(*
xml 存n行，每行4个参数，bool-可用位vaild、bool-输出位状态、bool-正反向输出标记位、lreal-节点坐标
使用METH进行调用，以实现区分功能， 以及少点高速性能。运行一次最多8个点。
.RUN() 一次加载全部数据，不支持中途改值
*)

FUNCTION_BLOCK FB_EL5131_SingleCycle
VAR CONSTANT
	{attribute 'displaymode':='hex'}
	cMaxCounterValue										: 	UDINT := 4294967295;
END_VAR
VAR_INPUT
	{attribute 'hide'} // 尝试隐藏该变量
	nDistWindow												:	UINT := 5;
	stEl5131												:	REFERENCE TO ST_EL5131;
	rScaleFactor      										: 	LREAL := 1; // 分子/分母
	{attribute 'displaymode':='bin'}
	OutputOption											:	USINT := 2#0000_0001; // chn 1 output
	InputOption												:	REFERENCE TO ST_EL5131_Setting;
END_VAR
VAR_OUTPUT
	bBusy													:	BOOL;
	bDone													:	BOOL;
	bError													:	BOOL;
	nErrId													:	UDINT;
	sErr													:	STRING;
	bInited													:	BOOL;
END_VAR
VAR
	{attribute 'hide'}
	_nMem													:	WORD;// bit 0 / 1 /2
	{attribute 'hide'}
	_pControOutput											:	POINTER TO ST_ENC_Control_Output_Channel;
	{attribute 'hide'}
	i														:	INT;
	{attribute 'hide'}
	_CamData												:	FB_MEM_TO_DATA_ST_EL5131_CamData;	
	{attribute 'hide'}
	_nNum													:	USINT;
	{attribute 'hide'}
	_tLastDurationDelay										:	TON :=(PT:= T#0S);
	{attribute 'hide'}
	nLastCounterValue										:	UDINT;
	{attribute 'hide'}
	_nTempLint												:	LINT;
	{attribute 'hide'}
	bForward												:	BOOL;
	{attribute 'hide'}
	bBackward												:	BOOL;
END_VAR

METHOD Cyclic : BOOL
VAR_INPUT
END_VAR
IF NOT __ISVALIDREF(stEl5131)
THEN
	RETURN;
END_IF
IF NOT _nMem.2
THEN 
	_nMem.2											:= TRUE;
	nLastCounterValue								:= stEl5131.PdoToPlc.Counter_value;
END_IF
bForward											:= FALSE;
bBackward											:= FALSE;
IF nLastCounterValue <> stEl5131.PdoToPlc.Counter_value
THEN 
	IF stEl5131.PdoToPlc.Counter_value > nLastCounterValue
	THEN 
		bForward									:= TRUE;
		bBackward									:= FALSE;
	END_IF
	IF stEl5131.PdoToPlc.Counter_value < nLastCounterValue
	THEN 
		bForward									:= FALSE;
		bBackward									:= TRUE;
	END_IF
	
	nLastCounterValue								:= stEl5131.PdoToPlc.Counter_value;
END_IF
END_METHOD

METHOD Init : BOOL
VAR_INPUT
	bExecute		:	BOOL;
END_VAR
Init														:= TRUE;
bInited														:= FALSE;
IF bExecute 
THEN
	IF NOT __ISVALIDREF(stEl5131)
	OR NOT (OutputOption.0 OR OutputOption.1)
	OR NOT __ISVALIDREF(InputOption)
	THEN 
		bBusy 												:= FALSE;
		bDone												:= FALSE;
		bError												:= TRUE;
		nErrId.0											:= TRUE;
		sErr												:= 'FB_EL5131_SingleCycle | FB_INPUT is not valid';
		RETURN;
	END_IF

	bBusy 													:= FALSE;
	bDone													:= FALSE;
	bError													:= FALSE;
	nErrId													:= 0;
	sErr													:= '';
	_nMem													:= 0;
	IF OutputOption.0 
	THEN 
		_pControOutput 										:= ADR(stEl5131.PlcToPdo.Contro_OutputChn1);
	END_IF							
	IF NOT OutputOption.0 
	AND OutputOption.1
	THEN 
		_pControOutput 										:= ADR(stEl5131.PlcToPdo.Contro_OutputChn2);
	END_IF
	_pControOutput^.Control.Enable_thresholds_output		:= TRUE;
	_pControOutput^.Control.Disalbe_thresholds_ccw			:= TRUE; // 在RUN 中根据情况再给false
	_pControOutput^.Control.Disalbe_thresholds_cw			:= TRUE; // 在RUN 中根据情况再给false
	_pControOutput^.Control.Set_tristate					:= InputOption.SetTristate;
	bInited													:= TRUE;
	Init													:= FALSE;
	
END_IF
END_METHOD

// 禁止模块输出
METHOD Reset : BOOL
VAR_INPUT
	bExecute		:	BOOL;
END_VAR
Reset														:= TRUE;
IF bExecute 
THEN 
	IF NOT __ISVALIDREF(stEl5131)
	OR NOT (OutputOption.0 OR OutputOption.1)
	OR NOT __ISVALIDREF(InputOption)
	THEN 
		bBusy 												:= FALSE;
		bDone												:= FALSE;
		bError												:= TRUE;
		nErrId.0											:= TRUE;
		sErr												:= 'FB_EL5131_SingleCycle | FB_INPUT is not valid';
		RETURN;
	END_IF
	// reset
	bBusy 													:= FALSE;
	bDone													:= FALSE;
	bError													:= FALSE;
	nErrId													:= 0;
	sErr													:= '';
	_nMem													:= 0;
	IF OutputOption.0 
	THEN 
		_pControOutput 										:= ADR(stEl5131.PlcToPdo.Contro_OutputChn1);
	END_IF
	IF NOT OutputOption.0 
	AND OutputOption.1
	THEN 
		_pControOutput 										:= ADR(stEl5131.PlcToPdo.Contro_OutputChn2);
	END_IF
	_pControOutput^.Control.Enable_thresholds_output		:= FALSE;
	_pControOutput^.Control.Disalbe_thresholds_ccw			:= TRUE;
	_pControOutput^.Control.Disalbe_thresholds_cw			:= TRUE;
	_pControOutput^.Control.Set_tristate					:= InputOption.SetTristate;
	bInited													:= FALSE;
	Reset													:= FALSE;
END_IF
END_METHOD

METHOD Run : BOOL
VAR_INPUT
	bExecute												:	BOOL;
	pstEL5131_CamData										:	POINTER TO ST_EL5131_CamData;
	nSize													:	ULINT;
END_VAR
Run															:= TRUE;
IF bExecute 
THEN 
	IF NOT __ISVALIDREF(stEl5131)
	OR NOT (OutputOption.0 OR OutputOption.1)
	OR NOT __ISVALIDREF(InputOption)
	THEN 
		bBusy 												:= FALSE;
		bDone												:= FALSE;
		bError												:= TRUE;
		nErrId.0											:= TRUE;
		sErr												:= 'FB_EL5131_SingleCycle | FB_INPUT is not valid';
		RETURN;
	END_IF
	IF NOT bInited
	THEN
		bBusy 												:= FALSE;
		bDone												:= FALSE;
		bError												:= TRUE;
		nErrId.1											:= TRUE;
		sErr												:= 'FB_EL5131_SingleCycle is not inited';
		RETURN;
	END_IF
	_nNum													:= TO_USINT(nSize/16);
	IF NOT _nMem.1
	THEN 
		FOR i:=1 TO _nNum BY 1
		DO
			_pControOutput^.Output_state					:= TO_USINT(CSETBIT32(_pControOutput^.Output_state,
																		TO_SINT(i-1),_CamData.get_bOutputState(TO_UDINT(i),pstEL5131_CamData)));
			_pControOutput^.Threshold[i]					:= TO_UDINT(_CamData.get_rPos(TO_UDINT(i),pstEL5131_CamData) / rScaleFactor) MOD cMaxCounterValue;
			_pControOutput^.Duration[i]						:= _CamData.get_nDuration(TO_UDINT(i),pstEL5131_CamData);
			_pControOutput^.Control.Disalbe_thresholds_ccw	:= InputOption.DisableThresholdsCcw; 
			_pControOutput^.Control.Disalbe_thresholds_cw	:= InputOption.DisableThresholdsCw;
		END_FOR
		_pControOutput^.Number_of_output_events 			:= _nNum;
		_pControOutput^.Control.Enable_thresholds_output	:= TRUE;
		_nMem.1												:= TRUE;
	END_IF
	IF _nMem.1	
	THEN// 判断是否完成全部
		IF stEl5131.PdoToPlc.Counter_value >= _pControOutput^.Threshold[_nNum] AND bForward // 额外需要判断是正转
		AND _pControOutput^.Control.Disalbe_thresholds_ccw AND NOT _pControOutput^.Control.Disalbe_thresholds_cw 
		
		OR stEl5131.PdoToPlc.Counter_value <= _pControOutput^.Threshold[_nNum] AND bBackward // 额外需要判断是反转
		AND NOT _pControOutput^.Control.Disalbe_thresholds_ccw AND _pControOutput^.Control.Disalbe_thresholds_cw 
		THEN 
			IF _pControOutput^.Duration[_nNum] <> 0 // 等待最后一个延时到达
			THEN// 判断最后一个是否有延时
				_tLastDurationDelay(IN:= TRUE,PT:= TO_TIME(_pControOutput^.Duration[_nNum])/1000);// to_time unit=ms,Duration's unit=us
				IF _tLastDurationDelay.Q
				THEN// done
					Run										:= FALSE;
					_tLastDurationDelay(IN:= FALSE);
				END_IF
			ELSE
				Run											:= FALSE;
				_tLastDurationDelay(IN:= FALSE);
			END_IF
			
		END_IF
	END_IF

END_IF
END_METHOD

METHOD SetRefPos : BOOL
VAR_INPUT
	bExecute		:	BOOL;
	rRefPos			:	LREAL;
END_VAR
SetRefPos													:= TRUE;
IF bExecute 
THEN 
	IF NOT __ISVALIDREF(stEl5131)
	THEN
		RETURN;
	END_IF
	IF stEl5131.PdoToPlc.Status.Set_counter_done AND NOT _nMem.0
	THEN 
		stEl5131.PlcToPdo.Control.Set_counter				:= FALSE;
		_nMem.0												:= TRUE;
	ELSE
		
		IF NOT stEl5131.PdoToPlc.Status.Set_counter_done 
		THEN 
			stEl5131.PlcToPdo.Set_counter_value					:= TO_UDINT(rRefPos / rScaleFactor) MOD cMaxCounterValue;	
			stEl5131.PlcToPdo.Control.Set_counter				:= TRUE;
		ELSE 
			_nTempLint											:= ABS(TO_LINT(stEl5131.PdoToPlc.Counter_value)
																	- TO_LINT(stEl5131.PlcToPdo.Set_counter_value));
			IF  _nTempLint <= nDistWindow
			THEN 
				stEl5131.PlcToPdo.Control.Set_counter				:= FALSE;
				_nMem.0												:= FALSE;
				SetRefPos											:= FALSE;
			END_IF
	
		END_IF
	END_IF
END_IF
END_METHOD

END_FUNCTION_BLOCK
